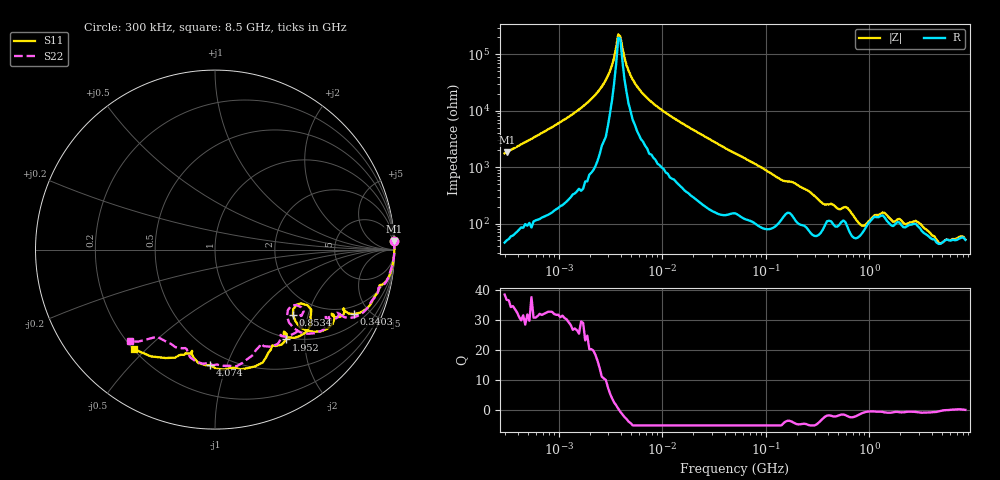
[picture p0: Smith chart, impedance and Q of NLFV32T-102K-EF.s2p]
! S-parameter Generated by TDK Corporation
! Copyright(C) 2015 TDK Corporation.
! All Rights Reserved.
! TDK P/N: NLFV32T-102K-EF (Inductors)
! Property: L=1000uH at 252kHz
! Size(LxWxT): 3.2x2.5x2.2mm, 0.126x0.098x0.087inches
! Model Type: s2p (Touchstone File Format Version 1.0)
! Frequency: DC=Yes Start=0.3MHz Stop=8500MHz 225points Log-sweep
! Note:
! Model Generated on Jun. 23, 2015
! Hash(MD5):
! Port Assignments:
!  1 ---@@@--- 2
! Applicable Conditions:
!  Temperature = 25 degC
!  DC Bias Current = 0 A
!  Small Signal Operation
! Terms and conditions regarding TDK Simulation Models
! (1)This simulation model is being provided solely for informational purposes. Please refer to the specifications of the products in terms of detailed characteristics of such products.
! (2)In no event shall TDK Corporation of any of its subsidiaries be liable for any loss or damage arising, directly or indirectly,
!  From any information contained in this simulation model, including, but not limited to loss or damages arising from any inaccuracies, omissions or errors in connection with such information.
! (3)Any and all copyrights on this simulation model are owned by TDK Corporation.
!  Duplication or redistribution of this simulation model without prior written permission from TDK Corporation is prohibited.
! (4)This simulation model is subject to any modification or change without any prior notice.
! (5)Neither TDK Corporation nor any of its subsidiaries shall make any warranty, express or implied,
!  Including but not limited to the correctness, implied warranties of merchantability and fitness for a particular purpose with respect to this simulation models.
! (6)The use of this simulation model shall be deemed to have consented to the terms and conditions hereof.
# MHz S MA R 50
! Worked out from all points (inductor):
!   224 points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, 300 kHz to 8.5 GHz, reference 50 ohm
!   read as one part in series: L = 923 uH near 314.1 kHz
!   highest Q = 36.7 at 314.1 kHz (marker M1), where L = 935 uH
!   self-resonance near 3.76 MHz
!   S11 on the Smith chart (normalised r, x): 300 kHz: 2, +39; 340.3 MHz: 1.52, -3.97; 853.4 MHz: 1.49, -1.61; 1.952 GHz: 0.96, -1.63; 4.074 GHz: 0.40, -0.88; 8.5 GHz: 0.20, -0.46
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0.3  0.9973 2.9  0.05659 -85.6  0.05717 -85.9  0.9966 2.9
0.3141136  0.9974 2.8  0.05403 -85.7  0.05453 -86.0  0.9969 2.7
1.72111  0.9996 0.4  0.00831 -87.7  0.00834 -88.1  0.9998 0.3
2.988094  0.9997 0.0  0.002392 -82.5  0.002399 -82.8  0.9997 -0.1
3.429973  0.9995 -0.0  0.001144 -69.4  0.001145 -70.3  0.9997 -0.2
3.760292  0.9995 -0.1  0.0004417 -29.5  0.0004362 -30.8  0.9997 -0.2
3.937196  0.9995 -0.1  0.000479 24.2  0.0004775 22.4  0.9996 -0.3
4.519427  0.9994 -0.2  0.001547 70.3  0.001541 70.1  0.9995 -0.3
5.187759  0.9995 -0.3  0.002778 78.6  0.002777 78.3  0.9994 -0.4
9.430415  0.9991 -0.7  0.009075 83.5  0.00907 83.2  0.9989 -0.9
51.67171  0.9939 -4.2  0.05735 80.6  0.05736 80.4  0.9915 -4.6
283.1228  0.9136 -20.3  0.2687 58.2  0.2689 58.0  0.9041 -21.9
340.2802  0.8515 -25.0  0.3392 48.1  0.3393 47.9  0.8403 -27.0
710.042  0.7144 -39.8  0.4773 26.7  0.4774 26.4  0.6983 -42.2
853.3868  0.5677 -40.1  0.5334 7.9  0.5339 7.6  0.5471 -42.8
1073.923  0.6007 -31.0  0.4242 -7.0  0.4235 -7.1  0.5788 -33.8
1551.304  0.6613 -48.0  0.4153 -1.7  0.4155 -2.3  0.6375 -48.1
1952.199  0.639 -51.6  0.4113 -12.2  0.4116 -12.4  0.631 -56.2
2819.992  0.6831 -67.1  0.3926 -24.4  0.3928 -24.9  0.6234 -69.9
4073.536  0.6451 -92.3  0.4617 -35.4  0.4639 -36.2  0.6346 -93.6
7072.242  0.6201 -108.5  0.3887 -82.0  0.39 -82.7  0.5819 -123.5
8500  0.715 -129.1  0.2789 -91.5  0.2784 -90.8  0.6985 -133.0
